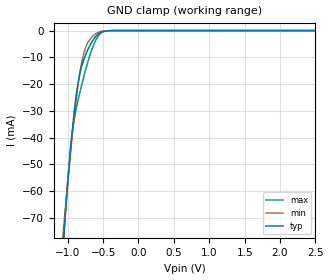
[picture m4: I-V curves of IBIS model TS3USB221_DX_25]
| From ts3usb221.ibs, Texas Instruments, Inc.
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[Model]   TS3USB221_DX_25
Model_type  Terminator
| variable   typ   min   max
C_comp   3.41pF   3.17pF   3.72pF
| C_tri-state   3.41pF   3.17pF   3.72pF
[Temperature Range]   40   100   -40
| Ambient temperature   25   85   -40
[Voltage range]   2.5   2.3   2.7
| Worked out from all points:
|   GND clamp passes 1 mA (typ) near -0.55 V on its own axis
[GND Clamp]
| TS3USB221_DX_25
|   Voltage   I(typ)   I(min)   I(max)
-2.5V     -720.6mA   -626.1mA   -808.2mA
-1.065V   -79.88mA   -76.09mA   -81.36mA
-1.04V    -71.02mA   -68.52mA   -71.25mA
-990mV    -54.17mA   -53.94mA   -52.95mA
-945mV    -40.39mA   -41.64mA   -40.17mA
-900mV    -28.62mA   -30.39mA   -31.94mA
-850mV    -19.01mA   -19.67mA   -25.59mA
-800mV    -13.1mA    -11.61mA   -20.06mA
-740mV    -8.626mA   -5.914mA   -14.02mA
-585mV    -1.69mA    -909.1uA   -2.688mA
-345mV    -7.227uA   -5.545uA   -3.587uA
2.5V      579.7pA    1.118nA    66.58pA
